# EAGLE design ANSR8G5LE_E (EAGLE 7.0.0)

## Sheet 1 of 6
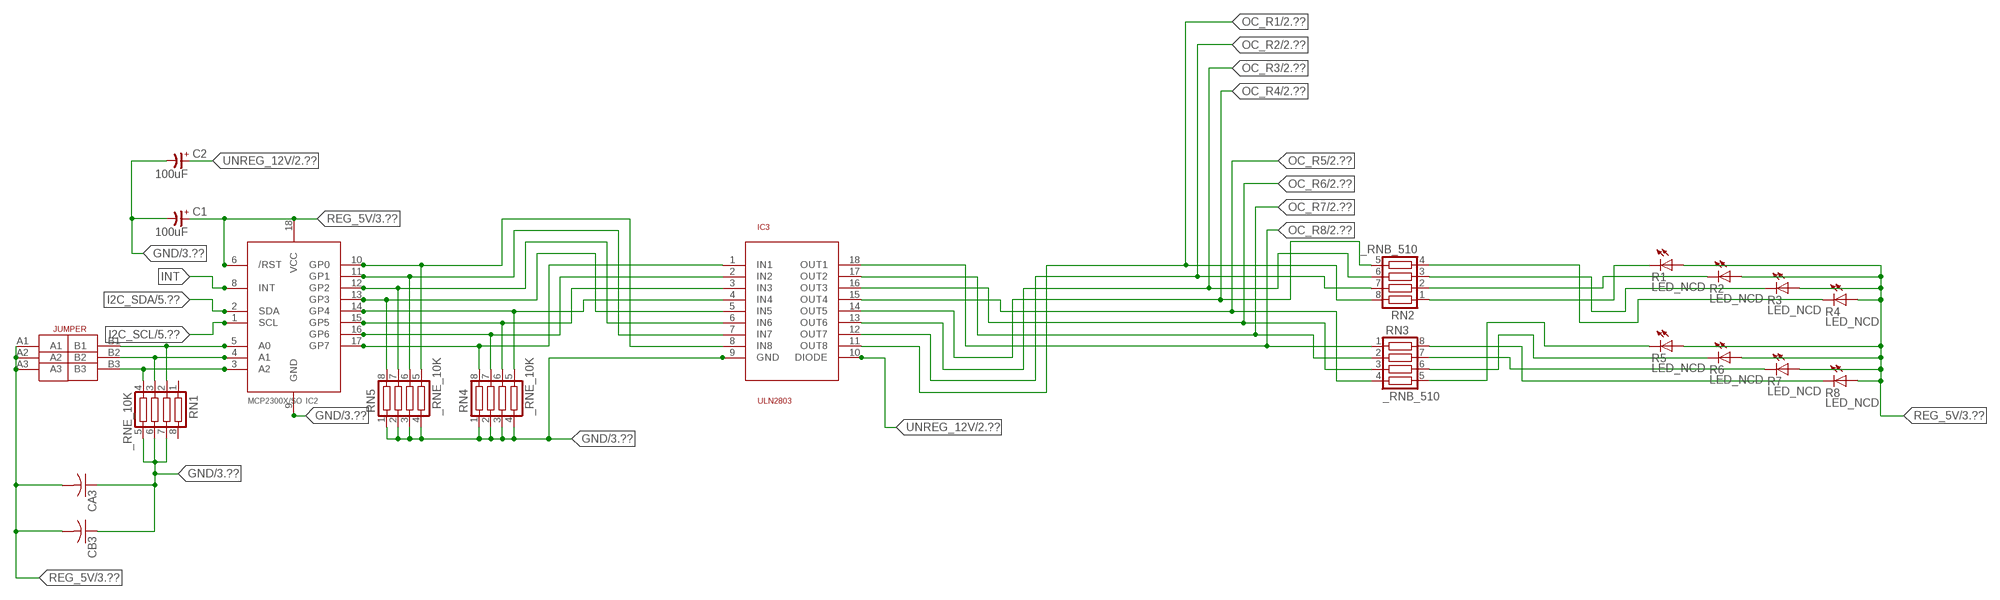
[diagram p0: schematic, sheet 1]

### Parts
C1  100uF  CP-E-025X060  [E-025X060]
C2  100uF  CP-E-025X060  [E-025X060]
CA3  CC1206KRX7R9BB104C1206K  [CC1206KRX7R9BB104]
CB3  TMK316F106ZL-TC1206K  [TMK316F106ZL-T]
IC2  MCP2300X/SO  [SO18W]
IC3  ULN2803  [SO18L]
R1  LED_NCD  [CHIPLED_0603]
R2  LED_NCD  [CHIPLED_0603]
R3  LED_NCD  [CHIPLED_0603]
R4  LED_NCD  [CHIPLED_0603]
R5  LED_NCD  [CHIPLED_0603]
R6  LED_NCD  [CHIPLED_0603]
R7  LED_NCD  [CHIPLED_0603]
R8  LED_NCD  [CHIPLED_0603]
RN1  _RNE_10K  [RNE]
RN2  _RNB_510  [RNB]
RN3  _RNB_510  [RNB]
RN4  _RNE_10K  [RNE]
RN5  _RNE_10K  [RNE]
U$18  JUMPER_3X2  [JUMPER_3X2]

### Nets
GND: C1.- C2.- CA3.1 CB3.1 IC2.9(GND) IC3.9(GND) RN1.5 RN1.6 RN1.7 RN4.1 RN4.2 RN4.3 RN4.4 RN5.1 RN5.2 RN5.3 RN5.4 ; also sheet 3,4,5,6
GP4: IC2.14(GP4) IC3.4(IN4) RN4.5
GP6: IC2.16(GP6) IC3.2(IN2) RN4.7
I2C_SCL: IC2.1(SCL) ; also sheet 5,6
I2C_SDA: IC2.2(SDA) ; also sheet 5,6
INT: IC2.8(INT)
N$6: IC2.5(A0) RN1.2 U$18.B1
N$7: IC2.4(A1) RN1.3 U$18.B2
N$8: IC2.3(A2) RN1.4 U$18.B3
N$20: R1.C RN2.1
N$21: IC2.12(GP2) IC3.6(IN6) RN5.7
N$22: IC2.11(GP1) IC3.7(IN7) RN5.6
N$23: IC2.10(GP0) IC3.8(IN8) RN5.5
N$29: R2.C RN2.2
N$30: R3.C RN2.3
N$31: R4.C RN2.4
N$32: R8.C RN3.8
N$81: R7.C RN3.7
N$82: R6.C RN3.6
N$83: R5.C RN3.5
N$89: IC2.13(GP3) IC3.5(IN5) RN5.8
N$93: IC2.15(GP5) IC3.3(IN3) RN4.6
N$94: IC2.17(GP7) IC3.1(IN1) RN4.8
OC_R1: IC3.11(OUT8) RN2.8 ; also sheet 2
OC_R2: IC3.12(OUT7) RN2.7 ; also sheet 2
OC_R3: IC3.13(OUT6) RN2.6 ; also sheet 2
OC_R4: IC3.14(OUT5) RN2.5 ; also sheet 2
OC_R5: IC3.15(OUT4) RN3.4 ; also sheet 2
OC_R6: IC3.16(OUT3) RN3.3 ; also sheet 2
OC_R7: IC3.17(OUT2) RN3.2 ; also sheet 2
OC_R8: IC3.18(OUT1) RN3.1 ; also sheet 2
REG_5V: C1.+ CA3.2 CB3.2 IC2.6(/RST) IC2.18(VCC) R1.A R2.A R3.A R4.A R5.A R6.A R7.A R8.A U$18.A1 U$18.A2 U$18.A3 ; also sheet 3,4,5,6
UNREG_12V: C2.+ IC3.10(DIODE) ; also sheet 2,3
Unconnected: RN1.1 RN1.8

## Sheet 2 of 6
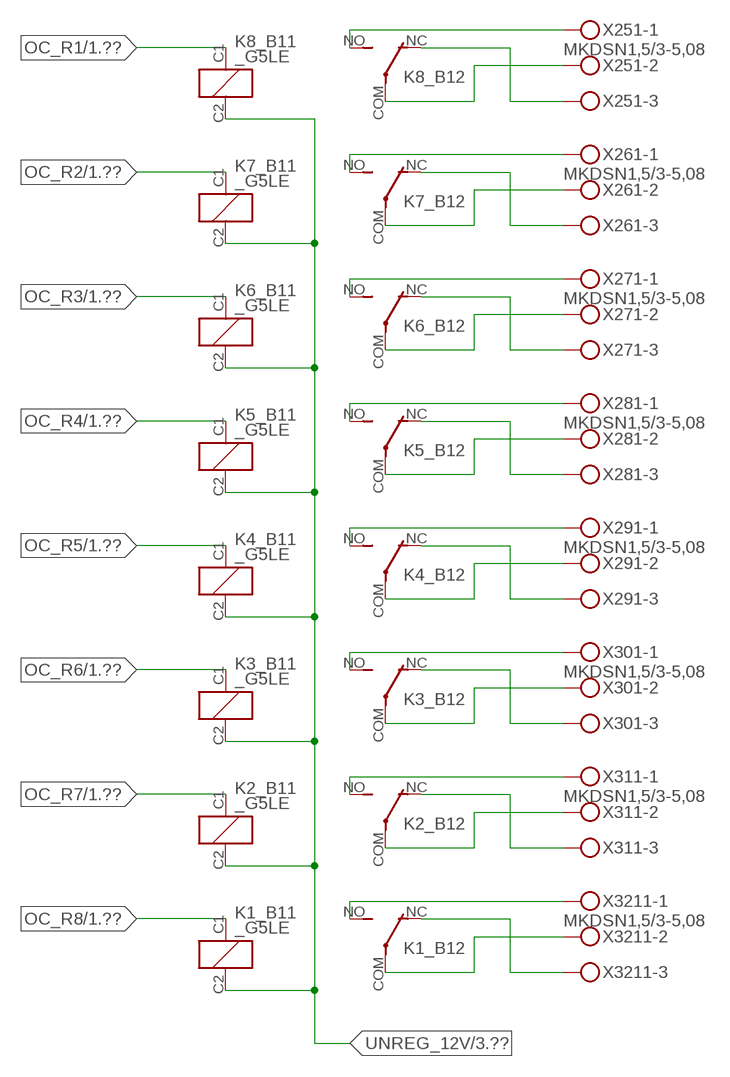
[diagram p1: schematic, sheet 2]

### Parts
K1_B1  _G5LE  [G5LE]
K2_B1  _G5LE  [G5LE]
K3_B1  _G5LE  [G5LE]
K4_B1  _G5LE  [G5LE]
K5_B1  _G5LE  [G5LE]
K6_B1  _G5LE  [G5LE]
K7_B1  _G5LE  [G5LE]
K8_B1  _G5LE  [G5LE]
X251  MKDSN1,5/3-5,08  [MKDSN1,5/3-5,08]
X261  MKDSN1,5/3-5,08  [MKDSN1,5/3-5,08]
X271  MKDSN1,5/3-5,08  [MKDSN1,5/3-5,08]
X281  MKDSN1,5/3-5,08  [MKDSN1,5/3-5,08]
X291  MKDSN1,5/3-5,08  [MKDSN1,5/3-5,08]
X301  MKDSN1,5/3-5,08  [MKDSN1,5/3-5,08]
X311  MKDSN1,5/3-5,08  [MKDSN1,5/3-5,08]
X3211  MKDSN1,5/3-5,08  [MKDSN1,5/3-5,08]

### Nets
N$203: K8_B1.COM(2:COM) X251.2
N$204: K8_B1.NC(2:NC) X251.3
N$205: K8_B1.NO(2:NO) X251.1
N$206: K7_B1.NO(2:NO) X261.1
N$207: K6_B1.NO(2:NO) X271.1
N$208: K7_B1.NC(2:NC) X261.3
N$209: K7_B1.COM(2:COM) X261.2
N$210: K6_B1.NC(2:NC) X271.3
N$211: K6_B1.COM(2:COM) X271.2
N$212: K5_B1.NC(2:NC) X281.3
N$213: K5_B1.COM(2:COM) X281.2
N$214: K5_B1.NO(2:NO) X281.1
N$215: K4_B1.NO(2:NO) X291.1
N$216: K4_B1.NC(2:NC) X291.3
N$217: K4_B1.COM(2:COM) X291.2
N$218: K3_B1.NO(2:NO) X301.1
N$219: K3_B1.NC(2:NC) X301.3
N$220: K3_B1.COM(2:COM) X301.2
N$221: K2_B1.NO(2:NO) X311.1
N$222: K2_B1.NC(2:NC) X311.3
N$223: K2_B1.COM(2:COM) X311.2
N$224: K1_B1.NO(2:NO) X3211.1
N$225: K1_B1.NC(2:NC) X3211.3
N$226: K1_B1.COM(2:COM) X3211.2
OC_R1: K8_B1.C1(1:C1) ; also sheet 1
OC_R2: K7_B1.C1(1:C1) ; also sheet 1
OC_R3: K6_B1.C1(1:C1) ; also sheet 1
OC_R4: K5_B1.C1(1:C1) ; also sheet 1
OC_R5: K4_B1.C1(1:C1) ; also sheet 1
OC_R6: K3_B1.C1(1:C1) ; also sheet 1
OC_R7: K2_B1.C1(1:C1) ; also sheet 1
OC_R8: K1_B1.C1(1:C1) ; also sheet 1
UNREG_12V: K1_B1.C2(1:C2) K2_B1.C2(1:C2) K3_B1.C2(1:C2) K4_B1.C2(1:C2) K5_B1.C2(1:C2) K6_B1.C2(1:C2) K7_B1.C2(1:C2) K8_B1.C2(1:C2) ; also sheet 1,3

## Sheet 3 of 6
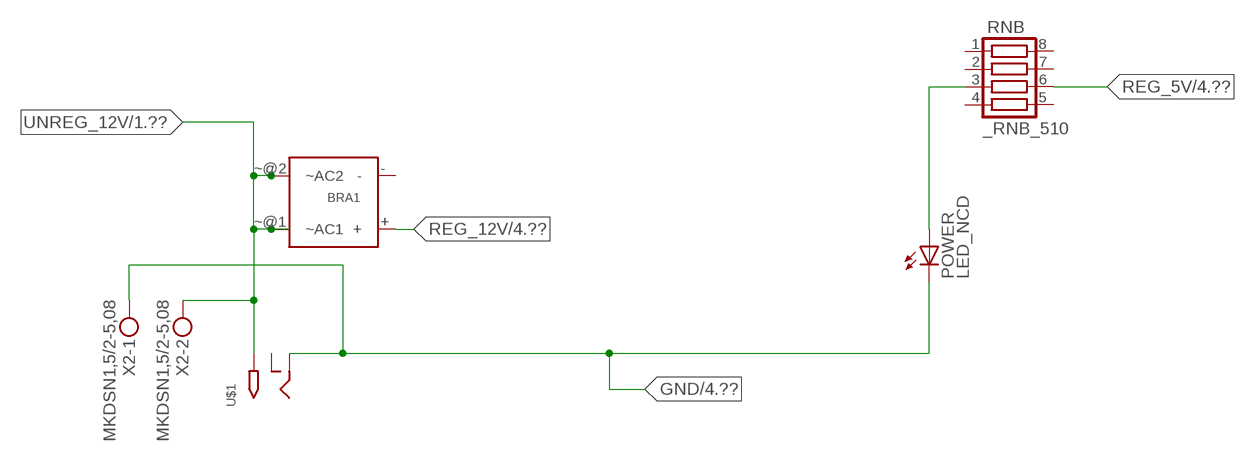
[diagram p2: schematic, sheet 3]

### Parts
BRA1  MB2S_  [MB2S]
POWER  LED_NCD  [CHIPLED_0603]
RNB  _RNB_510  [RNB]
U$1  2.1MMJACK  [PJ-102A]
X2  MKDSN1,5/2-5,08  [MKDSN1,5/2-5,08]

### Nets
GND: POWER.C U$1.RING X2.1 ; also sheet 1,4,5,6
N$2: POWER.A RNB.3
REG_5V: RNB.6 ; also sheet 1,4,5,6
REG_12V: BRA1.+ ; also sheet 4
UNREG_12V: BRA1.~@1(~AC1) BRA1.~@2(~AC2) U$1.TIP X2.2 ; also sheet 1,2
Unconnected: BRA1.- RNB.1 RNB.2 RNB.4 RNB.5 RNB.7 RNB.8 U$1.RING_SW

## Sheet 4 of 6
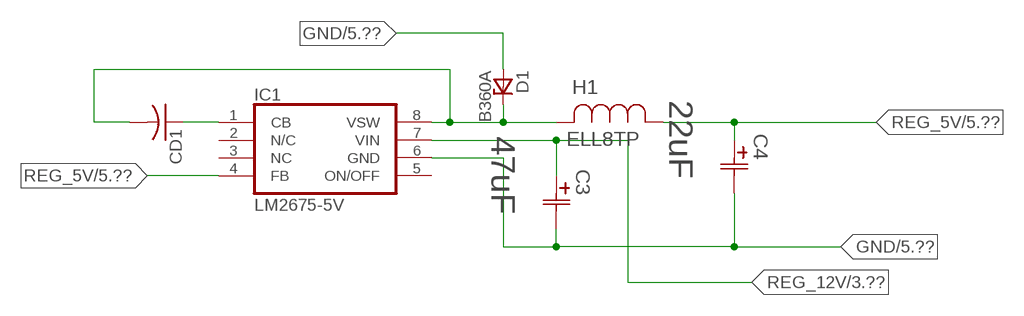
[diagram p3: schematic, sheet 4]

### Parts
C3  47uF  490-5463-6-NDCAP  [C2917(7343)-Y]
C4  22uF  490-5463-6-NDCAP  [C2917(7343)-Y]
CD1  _CD_10NF_50VC1206K  [_CD_10NF_50V]
D1  B360A  [DO214AC_ZENER]
H1  ELL8TP  [IND_ELL8TP]
IC1  LM2675-5V  LM2675  [SO-8]

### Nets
GND: C3.2(C2) C4.2(C2) D1.A IC1.6(GND) ; also sheet 1,3,5,6
N$1: CD1.2 D1.C H1.2 IC1.8(VSW)
N$3: CD1.1 IC1.1(CB)
REG_5V: C4.1(C1) H1.1 IC1.4(FB) ; also sheet 1,3,5,6
REG_12V: C3.1(C1) IC1.7(VIN) ; also sheet 3
Unconnected: IC1.2(N/C) IC1.5(ON/OFF)

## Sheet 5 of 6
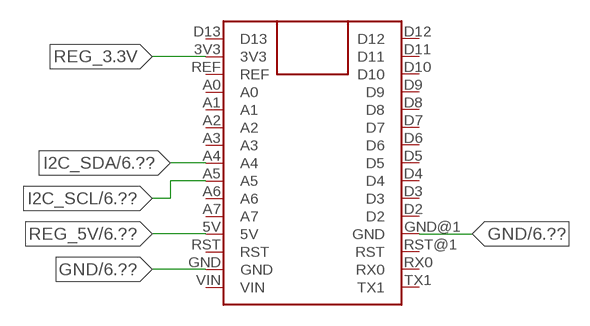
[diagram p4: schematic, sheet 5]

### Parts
FOR_NANO  ARDUINO_NANO  [ARDUINO_NANO]

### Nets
GND: FOR_NANO.GND FOR_NANO.GND@1(GND) ; also sheet 1,3,4,6
I2C_SCL: FOR_NANO.A5 ; also sheet 1,6
I2C_SDA: FOR_NANO.A4 ; also sheet 1,6
REG_3.3V: FOR_NANO.3V3
REG_5V: FOR_NANO.5V ; also sheet 1,3,4,6
Unconnected: FOR_NANO.A0 FOR_NANO.A1 FOR_NANO.A2 FOR_NANO.A3 FOR_NANO.A6 FOR_NANO.A7 FOR_NANO.D2 FOR_NANO.D3 FOR_NANO.D4 FOR_NANO.D5 FOR_NANO.D6 FOR_NANO.D7 FOR_NANO.D8 FOR_NANO.D9 FOR_NANO.D10 FOR_NANO.D11 FOR_NANO.D12 FOR_NANO.D13 FOR_NANO.REF FOR_NANO.RST FOR_NANO.RST@1(RST) FOR_NANO.RX0 FOR_NANO.TX1 FOR_NANO.VIN

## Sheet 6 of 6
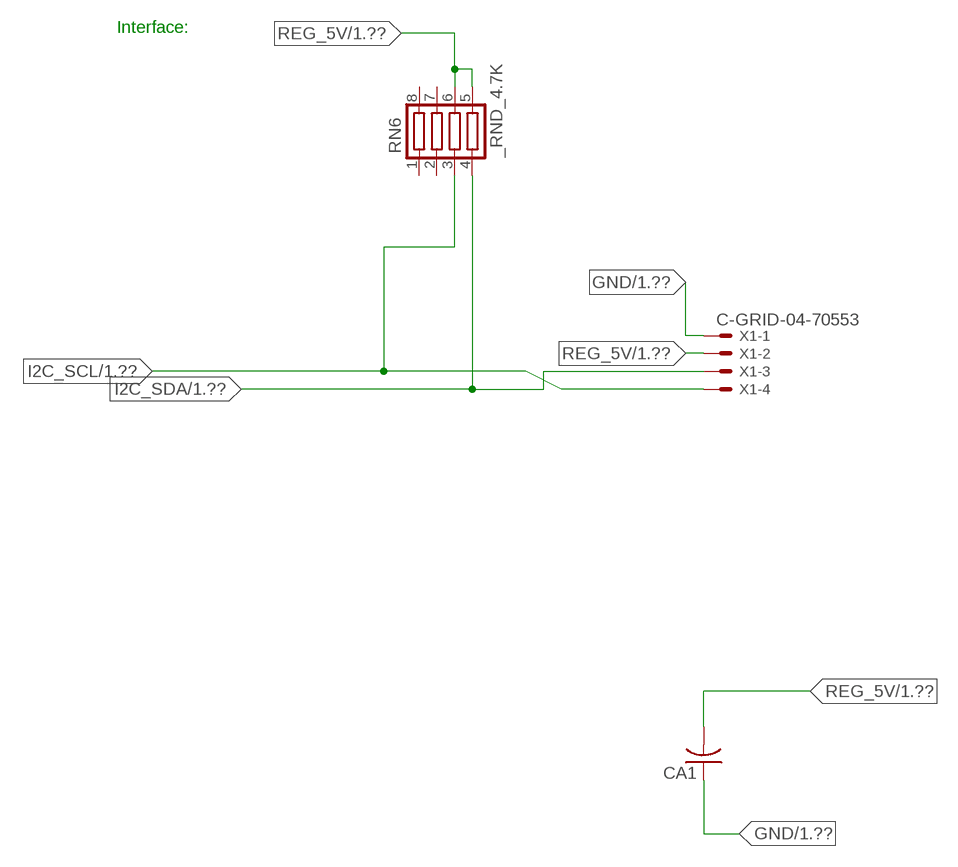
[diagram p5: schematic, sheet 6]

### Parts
CA1  CC1206KRX7R9BB104  [.1UF]
RN6  _RND_4.7K  [RND]
X1  C-GRID-04-70553  [70553-04]

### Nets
GND: CA1.1 X1.1 ; also sheet 1,3,4,5
I2C_SCL: RN6.3 X1.4 ; also sheet 1,5
I2C_SDA: RN6.4 X1.3 ; also sheet 1,5
REG_5V: CA1.2 RN6.5 RN6.6 X1.2 ; also sheet 1,3,4,5
Unconnected: RN6.1 RN6.2 RN6.7 RN6.8

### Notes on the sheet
- Interface:

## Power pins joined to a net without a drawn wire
NC: IC1.3(NC)

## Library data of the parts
BRA1 = NCD_ULTIMATE_LIBRARY:MB2S: Bridge Rectifier BRA MB2S 200V 500ma Digikey MB2S-TPMSTR-ND/MB2S-TP
C1 C2 = NCD_ULTIMATE_LIBRARY:CP-: Capacitors All Kinds POLARIZED CAP
C3 C4 = NCD_ULTIMATE_bhaskar:490-5463-6-ND: NCD CAP
CA1 CA3 = NCD_ULTIMATE_LIBRARY:CC1206KRX7R9BB104: Capacitor CA .1uF 50V SMT C1206K CC1206KRX7R9BB104
CB3 = NCD_ULTIMATE_LIBRARY:TMK316F106ZL-T: Capacitor CB 10uF SMT 1206 TMK316F106ZL-T
CD1 = NCD_ULTIMATE_LIBRARY:_CD_10NF_50V: Capacitor 10nF SMT
D1 = NCD_ULTIMATE_bhaskar:B360A: NCD DIODE B350A/B360A
FOR_NANO = NCD_ULTIMATE_CONNECTORS:ARDUINO_NANO
H1 = NCD_ULTIMATE_bhaskar:ELL8TP: NCD coil
IC1 = NCD_ULTIMATE_bhaskar:LM2675: LM2675 NCD http://www.ti.com/lit/ds/symlink/lm2675.pdf
IC2 = NCD_ULTIMATE_LIBRARY:MCP2300X: Semiconductor Port Expander I/O 8-Bit I2C MCP23008 Inexpensive i2c i/o expander - 8 general purpose i/o pins with optional pullups
IC3 = NCD_ULTIMATE_LIBRARY:ULN2803: Semiconductor 8 O.C. N-Channel Transistor Driver Digikey ULN2803AFWGCELTR-ND/ULN2803AFWG,C,EL
K1_B1 K2_B1 K3_B1 K4_B1 K5_B1 K6_B1 K7_B1 K8_B1 = NCD_ULTIMATE_LIBRARY:_G5LE: Relay 5A/10A SPDT; OC_FARNELL: unknown; OC_NEWARK: unknown
POWER = NCD_ULTIMATE_bhaskar:LED_NCD
R1-R8 = NCD_ULTIMATE_LIBRARY:LED_NCD: LED Digikey 754-1132-2-ND/APT2012SRCPRV
RN1 RN4 RN5 = NCD_ULTIMATE_LIBRARY:_RNE_10K: Resistor Array RNE SMT 10K x 4 Single Resistor Source: http://www.ctscorp.com/components/Datasheets/CTSChipArrayDs.pdf Digikey 742C083103JPTR-ND/742C083103JP; OC_FARNELL: unknown; OC_NEWARK: unknown
RN2 RN3 RNB = NCD_ULTIMATE_LIBRARY:_RNB_510: Resistor Array RNB SMT 510 x 4 Single Resistor Source: http://www.ctscorp.com/components/Datasheets/CTSChipArrayDs.pdf Digikey 742C083511JPTR-ND/ 742C083511JP; OC_FARNELL: unknown; OC_NEWARK: unknown
RN6 = NCD_ULTIMATE_LIBRARY:_RND_4.7K: Resistor Array RND SMT 4.7K x 4 Single Resistor Source: http://www.ctscorp.com/components/Datasheets/CTSChipArrayDs.pdf Digikey 742C083472JPTR-ND/742C083472JP; OC_FARNELL: unknown; OC_NEWARK: unknown
U$1 = NCD_ULTIMATE_CONNECTORS:2.1MMJACK: 2.1mm x 5.5mm DC jack with internal switch. Digikey part #PJ-102A, 4UCON part #05537 By microbuilder.eu
U$18 = NCD_ULTIMATE_CONNECTORS:JUMPER_3X2
X1 = NCD_ULTIMATE_CONNECTORS:C-GRID-04: CONNECTOR 4-Pos I2C wire to board 2.54 mm (0.100") pitch header Digikey WM1342-ND/0015912045; OC_FARNELL: unknown; OC_NEWARK: unknown
X2 = NCD_ULTIMATE_CONNECTORS:MKDSN1,5/2-5,08: MKDSN 1,5/ 2-5,08 Printklemme
X251 X261 X271 X281 X291 X301 X311 X3211 = NCD_ULTIMATE_CONNECTORS:MKDSN1,5/3-5,08: MKDSN 1,5/ 3-5,08 Printklemme Nennstrom: 13,5 A Nennspannung: 250 V Rastermaß: 5,08 mm Polzahl: 3 Anschlussart: Schraubanschluss Montage: Löten Anschlussrichtung Leiter/Platine: 0 ° Artikelnummer: 1729131 Source: http://eshop.phoenixcontact.com .. 1729131.pdf

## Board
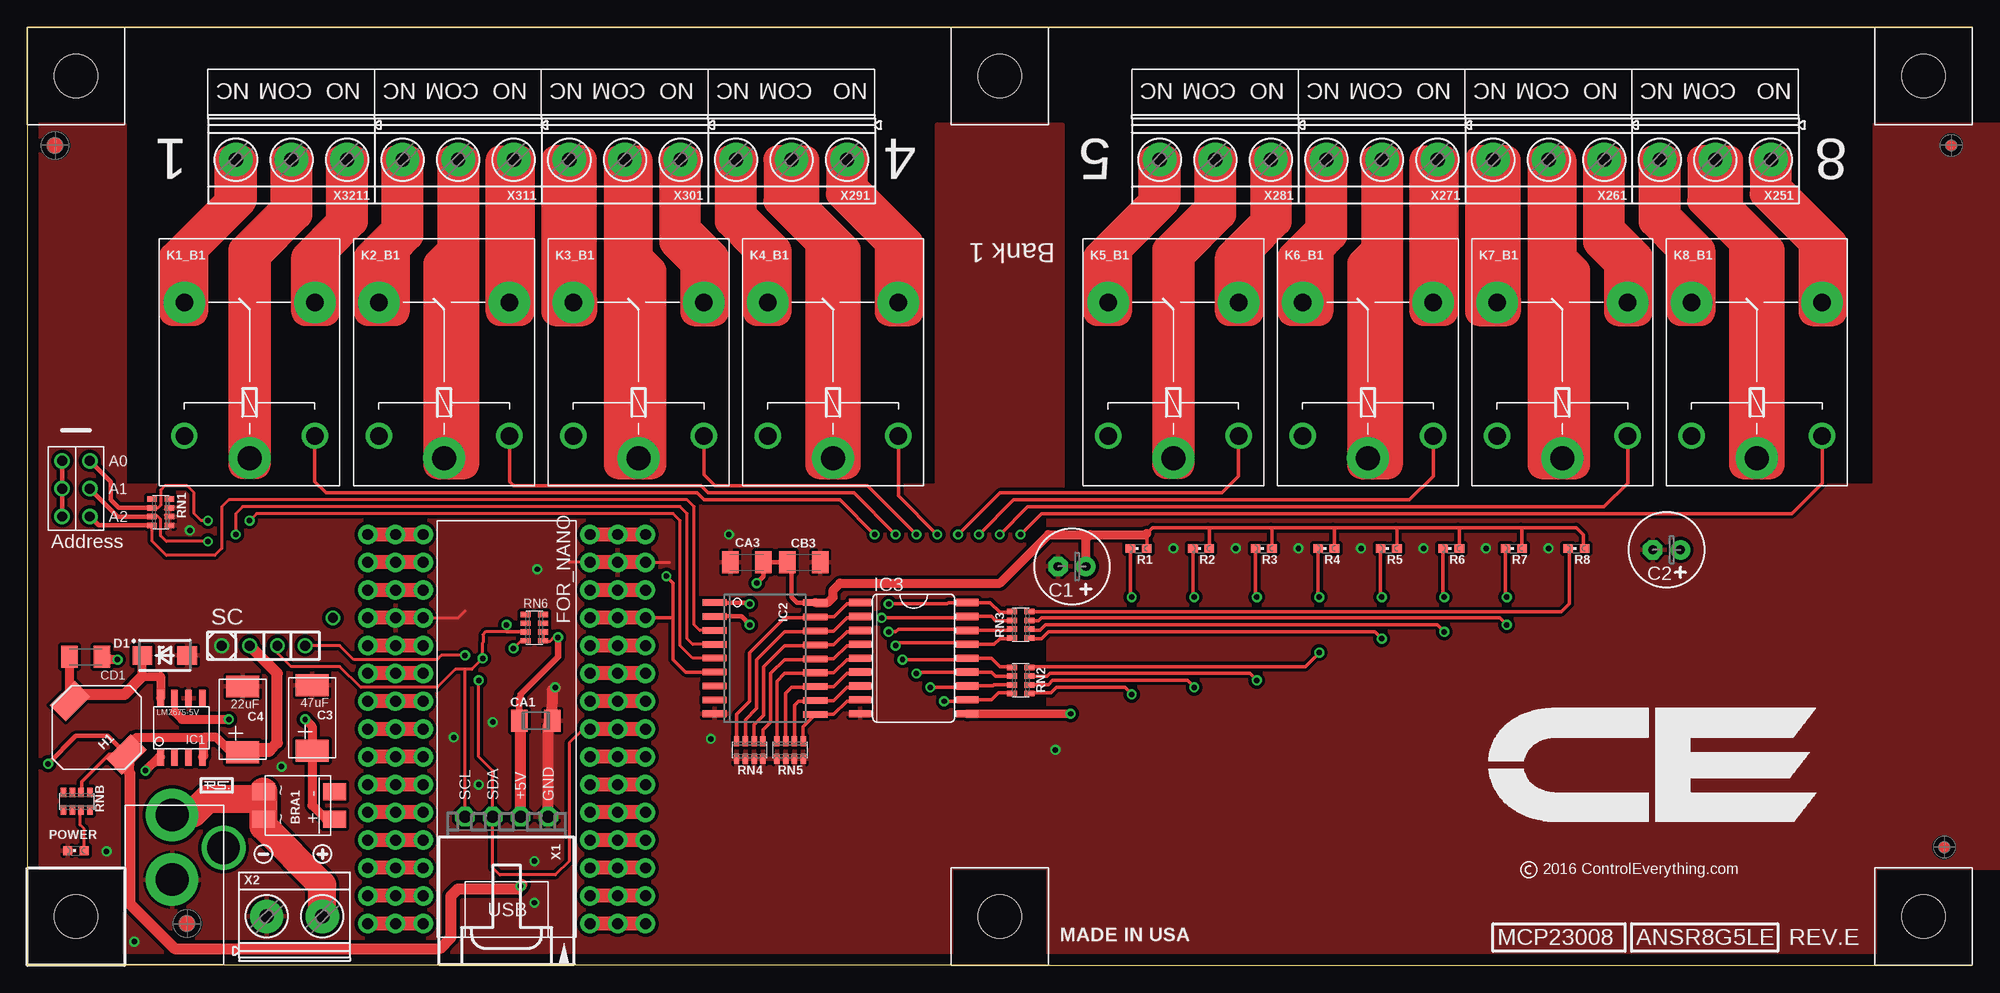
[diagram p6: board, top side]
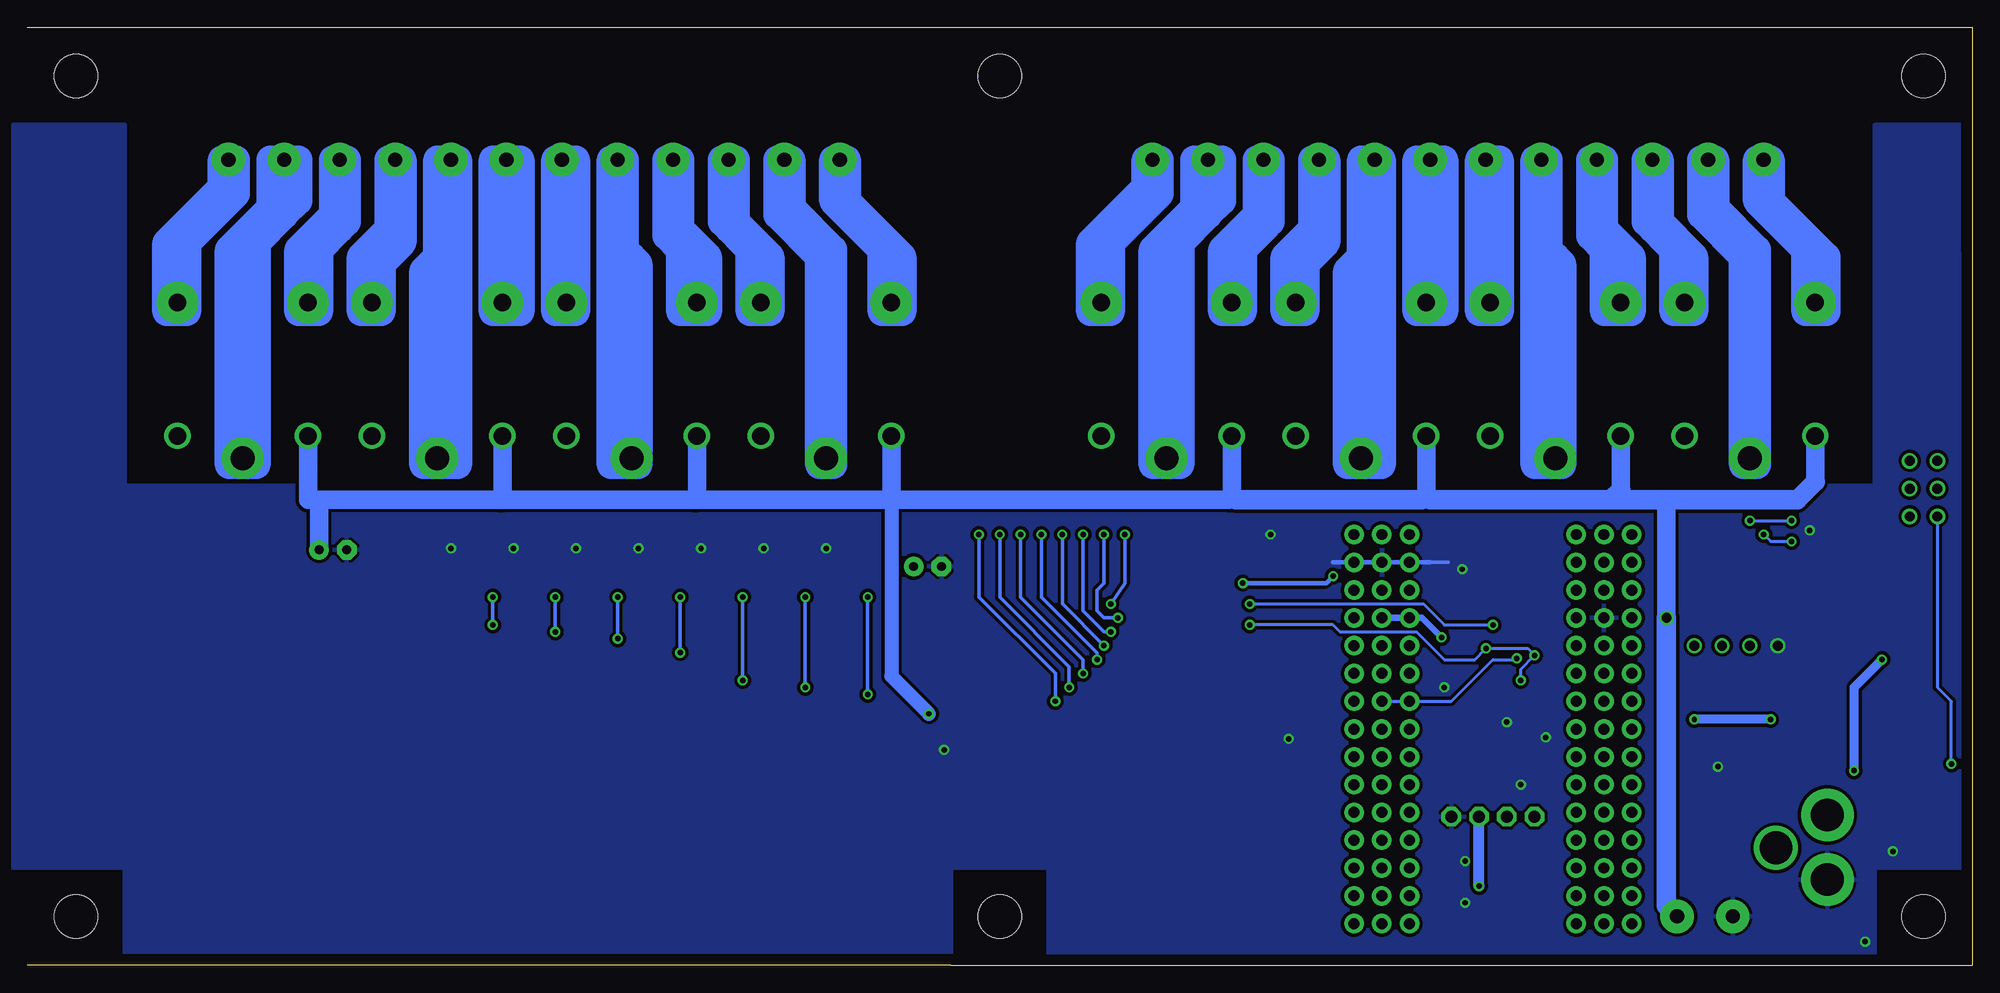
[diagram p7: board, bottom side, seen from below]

Size 177.8 x 85.73 mm. Coordinates in mm from the lower left corner, seen from the top.
Outline: 0,66.34 0,65.41
Outline: 0,65.41 0,0 93.34,0 177.8,0
Outline: 177.8,85.73 0,85.73 0,65.41
Copper layers (1*16): Top 0.035mm / dielectric 1.5mm / Bottom 0.035mm
Design rules "default": minimum track width 10mil, minimum drill 24mil, track to track 8mil, track to pad 8mil, pad to pad 8mil, via to via 8mil, smd to smd 8mil, copper to edge 40mil, drill to drill 8mil, minimum pad ring 10mil, minimum via ring 8mil, stop-mask expansion 4mil, vias tented up to drill 0mil, thermal gap 10mil
Holes 3.96 mm at 4.45,4.45 4.45,4.45 4.45,4.45 4.45,4.45

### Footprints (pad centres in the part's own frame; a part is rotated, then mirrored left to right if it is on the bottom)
MB2S = smd 1.55 x 2.1: + 0,-6.5; - 2.54,-6.5; ~@1 0,0; ~@2 2.54,0
E-025X060 = drill 0.813 pad 1.778: + -1.27,0 | drill 0.813 pad 1.778 octagon: - 1.27,0
C2917(7343)-Y = smd 2 x 3: 1 -3,0; 2 3,0
.1UF = smd 1.5 x 2: 1 -1.5,0; 2 1.5,0
CC1206KRX7R9BB104 = smd 1.5 x 2: 1 -1.5,0; 2 1.5,0
TMK316F106ZL-T = smd 1.5 x 2: 1 -1.5,0; 2 1.5,0
_CD_10NF_50V = smd 1.5 x 2: 1 -1.5,0; 2 1.5,0
DO214AC_ZENER = smd 1.8 x 1.7: A 2.05,0; C -2.05,0
ARDUINO_NANO = drill 1 pad 1.778: 3V1 -2.54,-2.54; 3V3 0,-2.54; 5V 0,-27.94; 5V1 -2.54,-27.94; A0 0,-7.62; A1 0,-10.16; A2 0,-12.7; A3 0,-15.24; A4 0,-17.78; A5 0,-20.32; A6 0,-22.86; A7 0,-25.4; A8 -2.54,-7.62; A9 -2.54,-10.16; A10 -2.54,-12.7; A11 -2.54,-15.24; A12 -2.54,-17.78; A13 -2.54,-20.32; A14 -2.54,-22.86; A15 -2.54,-25.4; D1 -2.54,0; D2 20.32,-25.4; D3 20.32,-22.86; D4 20.32,-20.32; D5 20.32,-17.78; D6 20.32,-15.24; D7 20.32,-12.7; D8 20.32,-10.16; D9 20.32,-7.62; D10 20.32,-5.08; D11 20.32,-2.54; D12 20.32,0; D13 0,0; D14 22.86,0; D15 22.86,-2.54; D16 22.86,-5.08; D17 22.86,-7.62; D18 22.86,-10.16; D19 22.86,-12.7; D20 22.86,-15.24; D21 22.86,-17.78; D22 22.86,-20.32; D23 22.86,-22.86; D24 22.86,-25.4; GND 0,-33.02; GND1 -2.54,-33.02; GND@1 20.32,-27.94; GND@2 22.86,-27.94; P$16 2.54,0; P$17 2.54,-2.54; P$18 2.54,-5.08; P$19 2.54,-7.62; P$20 2.54,-10.16; P$21 2.54,-12.7; P$22 2.54,-15.24; P$23 2.54,-17.78; P$24 2.54,-20.32; P$25 2.54,-22.86; P$26 2.54,-25.4; P$27 2.54,-27.94; P$28 2.54,-30.48; P$29 2.54,-33.02; P$30 2.54,-35.56; P$31 17.78,0; P$32 17.78,-2.54; P$33 17.78,-5.08; P$34 17.78,-7.62; P$35 17.78,-10.16; P$36 17.78,-12.7; P$37 17.78,-15.24; P$38 17.78,-17.78; P$39 17.78,-20.32; P$40 17.78,-22.86; P$41 17.78,-25.4; P$42 17.78,-27.94; P$43 17.78,-30.48; P$44 17.78,-33.02; P$45 17.78,-35.56; REF 0,-5.08; REF1 -2.54,-5.08; RST 0,-30.48; RST1 -2.54,-30.48; RST@1 20.32,-30.48; RST@2 22.86,-30.48; RX0 20.32,-33.02; RX1 22.86,-33.02; TX1 20.32,-35.56; TX2 22.86,-35.56; VIN 0,-35.56; VIN1 -2.54,-35.56
IND_ELL8TP = smd 2.054 x 3.2 rotated 45: 1 -2.442,-2.696; 2 2.442,2.442
SO-8 = smd 0.6 x 1.55: 1 -1.905,-2.69; 2 -0.635,-2.69; 3 0.635,-2.69; 4 1.905,-2.69; 5 1.905,2.71; 6 0.635,2.71; 7 -0.635,2.71; 8 -1.905,2.71
SO18W = smd 0.6 x 2.2: 1 -4.445,-4.6; 2 -3.175,-4.6; 3 -1.905,-4.6; 4 -0.635,-4.6; 5 0.635,-4.6; 6 1.905,-4.6; 7 3.175,-4.6; 8 4.445,-4.6; 9 5.715,-4.6; 10 5.775,4.6; 11 4.505,4.6; 12 3.235,4.6; 13 1.965,4.6; 14 0.695,4.6; 15 -0.575,4.6; 16 -1.845,4.6; 17 -3.145,4.6; 18 -4.445,4.6
SO18L = smd 0.66 x 2.032: 1 -5.08,-4.902; 2 -3.81,-4.902; 3 -2.54,-4.902; 4 -1.27,-4.902; 5 0,-4.902; 6 1.27,-4.902; 7 2.54,-4.902; 8 3.81,-4.902; 9 5.08,-4.902; 10 5.08,4.902; 11 3.81,4.902; 12 2.54,4.902; 13 1.27,4.902; 14 0,4.902; 15 -1.27,4.902; 16 -2.54,4.902; 17 -3.81,4.902; 18 -5.08,4.902
G5LE = drill 1.6: C1 -7.493,-5.969; C2 -7.493,5.969 | drill 2.2 pad 3.81: COM -9.525,0 | drill 1.6 pad 3.81: NC 4.699,5.969; NO 4.699,-5.969
CHIPLED_0603 = smd 0.8 x 0.8: A 0,-0.75; C 0,0.75
CHIPLED_0603' = smd 0.8 x 0.876: A 0,-0.75; C 0,0.75
RNE = smd 0.5 x 0.9: 1 -1.2,-0.8; 2 -0.4,-0.8; 3 0.4,-0.8; 4 1.2,-0.8; 5 1.2,0.8; 6 0.4,0.8; 7 -0.4,0.8; 8 -1.2,0.8
RNB = smd 0.5 x 0.9: 1 -1.2,-0.8; 2 -0.4,-0.8; 3 0.4,-0.8; 4 1.2,-0.8; 5 1.2,0.8; 6 0.4,0.8; 7 -0.4,0.8; 8 -1.2,0.8
RND = smd 0.5 x 0.9: 1 -1.2,-0.8; 2 -0.4,-0.8; 3 0.4,-0.8; 4 1.2,-0.8; 5 1.2,0.8; 6 0.4,0.8; 7 -0.4,0.8; 8 -1.2,0.8
PJ-102A = drill 3 pad 4.8: RING 0.1,-3.39; TIP 0.1,-9.29 | drill 3 pad 3.251: RING_SW -4.6,-6.29
PCB_MOUNTING_HOLE = hole 3.962: 4.445,4.445
JUMPER_3X2 = drill 0.9: A1 0,5.08; A2 0,2.54; A3 0,0; B1 2.54,5.08; B2 2.54,2.54; B3 2.54,0
70553-04 = drill 1.1 pad 1.778 octagon: 1 -3.81,-7.62; 2 -1.27,-7.62; 3 1.27,-7.62; 4 3.81,-7.62
MKDSN1,5/2-5,08 = drill 1.3 pad 3.048: 1 -2.561,0.025; 2 2.519,0.025
MKDSN1,5/3-5,08 = drill 1.3 pad 3.048: 1 -7.641,0.025; 2 -2.561,0.025; 3 2.519,0.025

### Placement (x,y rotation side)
BRA1  21.59,13.34 90 top
C1  95.5,36.45 180 top
C2  149.86,37.97 180 top
C3  26.04,22.61 90 top
C4  19.68,22.48 90 top
CA1  46.48,22.35 180 top
CA3  65.79,36.83 0 top
CB3  70.99,36.83 180 top
CD1  5.33,28.19 180 top
D1  12.57,28.32 0 top
FOR_NANO  53.98,3.81 180 top
H1  6.35,21.72 90 top
IC1  14.1,21.72 0 top
IC2  67.44,28.7 270 top
IC3  81.03,28.07 270 top
K1_B1  20.32,55.88 90 top
K2_B1  38.1,55.88 90 top
K3_B1  55.88,55.88 90 top
K4_B1  73.66,55.88 90 top
K5_B1  104.78,55.88 90 top
K6_B1  122.56,55.88 90 top
K7_B1  140.34,55.88 90 top
K8_B1  158.12,55.88 90 top
POWER  4.45,10.48 90 top
R1  LED_NCD  [CHIPLED_0603']  101.6,38.1 90 top
R2  LED_NCD  [CHIPLED_0603']  107.31,38.1 90 top
R3  LED_NCD  [CHIPLED_0603']  113.03,38.1 90 top
R4  LED_NCD  [CHIPLED_0603']  118.75,38.1 90 top
R5  LED_NCD  [CHIPLED_0603']  124.46,38.1 90 top
R6  LED_NCD  [CHIPLED_0603']  130.18,38.1 90 top
R7  LED_NCD  [CHIPLED_0603']  135.89,38.1 90 top
R8  LED_NCD  [CHIPLED_0603']  141.6,38.1 90 top
RN1  12.19,41.4 270 top
RN2  90.81,26.04 90 top
RN3  90.81,31.12 270 top
RN4  66.04,19.69 0 top
RN5  69.72,19.69 0 top
RN6  46.35,30.86 270 top
RNB  4.51,14.99 0 top
U$1  13.34,4.45 180 top
U$2  [VISION_REF15]  14.61,3.81 0 top
U$3  [ICON_MINUS]  21.59,10.16 180 top
U$4  [VISION_REF10]  175.26,10.79 270 top
U$5  PCB_MOUNTING_HOLE  [PCB_MOUNTING_HOLE]  177.8,76.84 90 top
U$6  PCB_MOUNTING_HOLE  [PCB_MOUNTING_HOLE]  93.34,0 90 top
U$7  PCB_MOUNTING_HOLE  [PCB_MOUNTING_HOLE]  93.34,76.84 90 top
U$8  PCB_MOUNTING_HOLE  [PCB_MOUNTING_HOLE]  8.89,76.84 90 top
U$9  [ICON_PLUS]  26.99,10.16 90 top
U$11  PCB_MOUNTING_HOLE  [PCB_MOUNTING_HOLE]  177.8,0 90 top
U$12  PCB_MOUNTING_HOLE  [PCB_MOUNTING_HOLE]  177.8,76.84 90 top
U$15  [VISION_REF15]  2.54,74.93 270 top
U$18  3.17,41.02 0 top
U$21  [ICON_USA]  94.36,2.16 0 top
U$28  [VISION_REF10]  175.9,74.93 270 top
X1  43.81,5.97 180 top
X2  24.45,4.45 0 top
X251  151.76,73.66 180 top
X261  136.53,73.66 180 top
X271  121.28,73.66 180 top
X281  106.05,73.66 180 top
X291  67.31,73.66 180 top
X301  52.07,73.66 180 top
X311  36.83,73.66 180 top
X3211  21.59,73.66 180 top

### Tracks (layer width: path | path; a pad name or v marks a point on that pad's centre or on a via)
GND  (via drill 0.5, 0.9)
  Top 0.254: 36.2,31.75 39.37,31.75 40.01,32.38 | FOR_NANO.GND@1 32.38,31.75 | 49.53,36.83 56.52,36.83 58.67,36.83
  Top 1.016: X1.1 47.62,22 CA1.1 47.98,22.5 48.01,25.15 v48.26,25.4
  Bottom 0.254: 51.44,36.83 FOR_NANO.GND
  Bottom 0.305: 47.88,36.83 49.53,36.83 51.44,36.83
  Bottom 0.406: 49.53,36.83 58.42,36.83
  other vias: 14.86,39.75 62.48,20.7 127.64,38.1 93.98,19.69 133.35,38.1 139.06,38.1 121.92,38.1 116.2,38.1 110.49,38.1 104.78,38.1 64.14,39.37 9.78,2.16 17.78,29.21 41.27,16.51 46.35,9.53 46.61,36.2 46.35,5.71 42.55,22.23 38.99,20.83 7.24,10.41 23.24,18.16
  pour Bottom (isolate 0.305): -1.27,8.89 8.89,8.89 8.89,0 84.45,0 84.45,8.89 94.61,8.89 94.61,76.84 83.19,76.84 83.19,43.81 8.89,43.81 8.89,76.84 -1.27,76.84
  pour Top (isolate 0.305): -2.54,8.89 8.89,8.89 8.89,0 84.45,0 84.45,8.89 94.61,8.89 94.61,76.84 83.19,76.84 83.19,43.81 8.89,43.81 8.89,76.84 -2.54,76.84
  pour Top (isolate 0.305): 93.34,43.81 168.91,43.81 168.91,76.84 180.97,76.84 180.97,8.89 168.91,8.89 168.91,0 93.34,0
  pour Bottom (isolate 0.305): 93.34,0 93.34,43.81 168.91,43.81 168.91,76.84 179.07,76.84 179.07,8.89 168.91,8.89 168.91,0
GP4
  Top 0.305: RN4.5 67.24,21.52 67.94,22.23 67.94,26.67 69.22,27.94 71.97,27.94 IC2.14 73.73,28.01 74.93,29.21 76,29.21 IC3.4
GP6
  Top 0.305: RN4.7 65.64,22.46 66.67,23.5 66.67,27.94 69.22,30.48 71.97,30.48 IC2.16 73.73,30.55 74.93,31.75 76,31.75 IC3.2
I2C_SCL  (via drill 0.5, 0.9)
  Top 0.254: 40.01,27.05 40.64,27.05 v41.64,28.05 41.64,29.48 41.66,29.5 41.66,30.23 41.89,30.46 RN6.3 45.54,30.48 43.81,30.48 v43.81,31.12 | 40.01,27.05 39.12,27.05 37.47,25.4 30.48,25.4 28.57,27.3 24.13,27.3 22.86,28.58 v22.86,29.21 | X1.4 40.01,27.05
  Top 0.406: IC2.1 65.91,33.15 v66.04,33.02
  Bottom 0.254: v66.04,33.02 50.16,33.02 48.26,31.12 v43.81,31.12 | v41.64,28.05 41.75,27.94 43.81,27.94 47.62,24.13 FOR_NANO.A5
I2C_SDA  (via drill 0.5, 0.9)
  Top 0.254: RN6.4 45.16,29.66 v44.45,28.96 | 40,28.33 v40.01,28.32 37.85,28.32 37.47,27.94 29.84,27.94 28.57,29.21 v25.4,29.21 | v41.27,26.04 41.27,19.05 42.55,17.78 X1.3 42.55,8.89 43.18,8.26 48.26,8.26 49.53,9.53 49.53,20.32 50.8,21.59 51.44,21.59
  Top 0.406: IC2.2 65.28,31.88 v66.04,31.12
  Bottom 0.254: v66.04,31.12 58.42,31.12 57.78,30.48 50.8,30.48 48.26,27.94 45.47,27.94 v44.45,28.96 40.64,28.96 v40.01,28.32 41.27,27.05 v41.27,26.04
N$1
  Top 0.813: H1.2 3.88,24.77 | D1.C 10.52,26.4 12.19,26.38 IC1.8 | CD1.2 3.83,24.15 4.45,24.77
  Top 1.016: 3.88,24.77 4.45,24.77 8.89,24.77 10.52,26.4
N$2
  Top 0.254: POWER.A 5.2,12.46 4.83,12.83 4.83,14.1 RNB.3
  Top 0.406: 4.95,14.14 RNB.3
N$3  (via drill 0.5)
  Top 0.813: IC1.1 12.04,19.03 v10.79,17.78 | v8.26,27.94 7.72,27.94 CD1.1
  Bottom 0.813: v10.79,17.78 10.79,25.4 v8.26,27.94
N$6  (via drill 0.5)
  Top 0.254: IC2.5 60.83,28.07 59.69,29.21 59.69,40.64 59.05,41.27 20.95,41.27 v20.32,40.64 | v16.51,40.64 15.88,40.64 15.24,41.27 15.24,43.18 14.61,43.81 12.57,43.81 12.19,43.43 12.19,42.04 11.94,41.78 11.41,41.78 RN1.2
  Top 0.406: RN1.2 8.36,41.8 7.62,42.55 7.62,44.2 U$18.B1
  Bottom 0.254: v20.32,40.64 v16.51,40.64
N$7  (via drill 0.5)
  Top 0.254: IC2.4 60.83,29.34 60.33,29.84 60.33,41.27 59.69,41.91 19.68,41.91 19.05,41.27 v19.05,39.37 | v16.51,38.73 12.7,38.73 12.19,39.24 12.19,40.77 11.94,41.02 11.41,41.02 RN1.3
  Top 0.406: RN1.3 8.27,41 U$18.B2
  Bottom 0.254: v19.05,39.37 18.41,38.73 v16.51,38.73
N$8
  Top 0.254: IC2.3 61.47,30.61 60.96,31.12 60.96,41.91 60.33,42.55 18.41,42.55 17.78,41.91 17.78,38.1 17.14,37.47 12.7,37.47 11.43,38.73 11.43,40.16 RN1.4
  Top 0.406: RN1.4 6.53,40.2 U$18.B3
N$9
  Top 2.54: 74.95,73.64 74.95,70.46 79.38,66.04 79.38,60.83 79.63,60.58
N$10
  Top 2.54: 64.79,73.64 64.79,68.56 67.31,66.04 67.31,60.96 67.69,60.58
N$11
  Top 2.54: 69.87,73.64 69.87,69.83 73.66,66.04 73.66,46.35
N$12
  Top 2.54: 59.71,73.64 59.71,66.02 61.59,64.14 61.59,60.83 61.85,60.58
N$13
  Top 2.54: 49.55,73.64 49.55,60.94 49.91,60.58
N$14
  Top 2.54: 54.63,73.64 54.63,47.6 55.88,46.35
N$15
  Top 2.54: 44.47,73.64 44.47,60.98 44.07,60.58
N$16
  Top 2.54: 34.31,73.64 34.31,66.7 32.38,64.77 32.38,60.83 32.13,60.58
N$17
  Top 2.54: 39.39,73.64 39.39,47.65 38.1,46.35
N$18
  Top 2.54: 29.23,73.64 29.23,67.97 26.67,65.41 26.67,60.96 26.29,60.58
N$19
  Top 2.54: 19.07,73.64 19.07,69.87 14.61,65.41 14.61,60.83 14.35,60.58
N$20  (via drill 0.5)
  Top 0.305: R1.C 100.85,33.77 v100.97,33.66 | v100.97,24.77 100.33,25.4 94.11,25.4 93.6,24.89 91.66,24.89 RN2.1
  Bottom 0.305: v100.97,33.66 v100.97,24.77
N$21
  Top 0.305: RN5.7 69.32,24.87 69.85,25.4 71.97,25.4 IC2.12 73.73,25.47 74.93,26.67 76,26.67 IC3.6
N$22
  Top 0.305: RN5.6 70.12,23.77 70.48,24.13 71.97,24.13 IC2.11 73.73,24.2 74.93,25.4 76,25.4 IC3.7
N$23
  Top 0.254: 71.97,22.86 IC2.10
  Top 0.305: RN5.5 70.92,21.81 IC2.10 73.73,22.93 74.93,24.13 76,24.13 IC3.8
N$24
  Top 2.54: 24.15,73.64 24.15,69.24 20.32,65.41 20.32,46.35
N$25
  Bottom 2.54: 20.32,46.35 20.32,64.77 24.13,68.58 24.13,73.61 24.15,73.64
N$26
  Bottom 2.54: 14.35,60.58 14.35,65.15 19.05,69.85 19.05,73.61 19.07,73.64
N$27
  Bottom 2.54: 26.29,60.58 26.29,64.39 29.21,67.31 29.21,73.61 29.23,73.64
N$28
  Bottom 2.54: 44.07,60.58 44.07,63.12 44.45,63.5 44.45,73.61 44.47,73.64
N$29  (via drill 0.5)
  Top 0.305: R2.C 106.56,33.77 v106.68,33.66 | v106.68,25.4 106.05,26.04 93.73,26.04 93.34,25.65 91.62,25.65 RN2.2
  Bottom 0.305: v106.68,33.66 v106.68,25.4
N$30  (via drill 0.5)
  Top 0.305: R3.C 112.28,33.77 v112.39,33.66 | v112.39,26.04 111.76,26.67 93.47,26.67 93.22,26.42 91.62,26.42 RN2.3
  Bottom 0.305: v112.39,33.66 v112.39,26.04
N$31  (via drill 0.5)
  Top 0.305: R4.C 118,33.77 v118.11,33.66 | v118.11,28.58 116.84,27.3 91.67,27.3 RN2.4
  Bottom 0.305: v118.11,33.66 v118.11,28.58
N$32
  Top 0.305: RN3.8 140.26,32.31 140.97,33.02 140.97,37.98 R8.C
N$42
  Bottom 2.54: 61.85,60.58 61.85,63.88 59.69,66.04 59.69,73.61 59.71,73.64
N$43
  Bottom 2.54: 32.13,60.58 32.13,63.88 34.29,66.04 34.29,73.61 34.31,73.64
N$44
  Bottom 2.54: 38.1,46.35 38.1,64.77 39.37,66.04 39.37,73.61 39.39,73.64
N$45
  Bottom 2.54: 49.91,60.58 49.91,63.12 49.53,63.5 49.53,72.34 49.55,73.64
N$46
  Top 2.54: 49.53,62.87 49.53,73.66 50.16,73.66 50.16,62.87 | 49.53,62.87 50.16,62.87 | 50.16,62.87 50.16,62.23 | 50.16,62.23 50.16,60.32 49.53,60.32 49.53,60.96 | 49.53,60.96 49.53,62.23 | 49.53,62.87 49.53,62.23 | 49.53,62.23 50.16,62.23 | 49.53,60.96 50.8,60.96 | 50.8,60.96 50.8,73.66 48.26,73.66 48.26,59.69 50.8,59.69 50.8,60.96
N$47
  Bottom 2.54: 54.61,73.61 54.63,73.64
N$48
  Bottom 2.54: 55.88,46.35 55.88,63.5 54.61,64.77
N$49
  Top 2.54: 54.61,73.66 54.61,64.77 | 55.88,63.5 55.88,46.35 | 54.61,73.66 55.88,73.66 55.88,64.77 | 55.88,64.77 55.88,63.5 | 55.88,63.5 54.61,64.77 | 54.61,64.77 54.61,45.72 | 54.61,45.72 57.15,45.72 57.15,63.5 55.88,64.77 | 54.61,73.66 53.98,73.66 53.98,45.72 54.61,45.72
N$50
  Top 2.54: 59.05,66.67 59.05,73.66 60.33,73.66 60.33,67.31 62.87,64.77 62.87,59.69 60.96,59.69 60.96,64.14 | 59.05,66.67 60.96,64.77 60.96,64.14 | 59.05,66.67 59.05,66.04 60.96,64.14
N$51
  Top 2.54: 66.67,59.69 66.67,65.41 64.14,67.95 64.14,73.66 65.41,73.66 65.41,68.58 68.58,65.41 68.58,59.69 66.67,59.69
N$52
  Top 2.54: 69.85,73.66 68.58,73.66 68.58,69.85 71.12,67.31 | 71.12,67.31 72.39,66.04 72.39,45.72 74.93,45.72 74.93,64.77 | 74.93,64.77 69.85,69.85 69.85,73.66 | 69.85,73.66 71.12,73.66 71.12,69.22 | 71.12,69.22 71.12,67.31 | 74.93,64.77 74.93,65.41 71.12,69.22
N$53
  Top 2.54: 74.3,73.66 74.3,70.48 78.74,66.04 78.74,59.69 80.64,59.69 80.64,66.04 75.56,71.12 75.56,73.66 74.3,73.66
N$54
  Top 2.54: 45.09,73.66 45.09,59.69 43.18,59.69 43.18,73.66 45.09,73.66
N$55
  Top 2.54: 40.01,73.66 40.01,45.72 37.47,45.72 37.47,64.14 38.73,65.41 38.73,73.66 40.01,73.66
N$56
  Top 2.54: 34.92,73.66 34.92,66.67 33.66,65.41 33.66,59.69 31.11,59.69 31.11,64.77 33.66,67.31 33.66,73.66 34.92,73.66
N$57
  Top 2.54: 29.21,73.66 29.84,73.66 29.84,67.95 27.3,65.41 27.3,59.69 25.4,59.69 25.4,64.77 28.57,67.95 | 29.21,68.58 29.21,73.66 | 29.21,73.66 28.57,73.66 28.57,67.31
N$58
  Top 2.54: 24.77,69.22 24.77,73.66 24.13,73.66 | 24.77,69.22 23.5,67.95 | 23.5,67.95 20.95,65.41 20.95,64.77 | 20.95,64.77 20.95,45.72 19.68,45.72 19.68,65.41 24.13,69.85 24.13,73.66 | 24.13,73.66 23.5,73.66 23.5,67.95 | 24.77,69.22 24.77,68.58 20.95,64.77
N$59
  Top 2.54: 19.68,73.66 19.68,69.85 15.24,65.41 15.24,59.69 13.34,59.69 13.34,64.77 18.41,69.85 18.41,73.66 19.68,73.66
N$60
  Bottom 2.54: 19.05,73.66 18.41,73.66 18.41,69.85 13.34,64.77 13.34,59.69 15.24,59.69 15.24,65.41 19.68,69.85 19.68,73.66
N$61
  Bottom 2.54: 23.5,73.66 23.5,69.22 19.68,65.41 19.68,45.72 20.95,45.72 20.95,64.77 24.77,68.58 24.77,73.66 23.5,73.66
N$62
  Bottom 2.54: 28.57,73.66 28.57,67.95 25.4,64.77 25.4,59.69 27.3,59.69 27.3,65.41 29.84,67.95 29.84,73.66 28.57,73.66
N$63
  Bottom 2.54: 33.66,73.66 33.66,67.31 31.11,64.77 31.11,59.69 33.66,59.69 33.66,65.41 34.92,66.67 34.92,73.66 33.66,73.66
N$64
  Bottom 2.54: 38.73,73.66 38.73,65.41 37.47,64.14 37.47,45.72 40.01,45.72 40.01,73.66 38.73,73.66
N$65
  Bottom 2.54: 45.09,73.66 43.18,73.66 43.18,59.69 45.09,59.69 45.09,73.66
N$66
  Bottom 2.54: 48.26,73.66 48.26,59.69 50.8,59.69 50.8,73.66 48.26,73.66
N$67
  Bottom 2.54: 53.98,73.66 53.98,45.72 57.15,45.72 57.15,63.5 55.88,64.77 55.88,73.66 53.98,73.66
N$68
  Bottom 2.54: 59.05,73.66 59.05,66.04 60.96,64.14 60.96,59.69 62.87,59.69 62.87,64.77 60.33,67.31 60.33,73.66 59.05,73.66
N$69
  Bottom 2.54: 67.69,60.58 67.69,64.39 66.67,65.41 | 66.67,65.41 64.77,67.31 | 64.77,67.31 64.77,73.61 64.79,73.64 | 64.77,67.31 64.14,67.95 64.14,73.66 65.41,73.66 65.41,68.58 68.58,65.41 68.58,59.69 66.67,59.69 66.67,65.41
N$70
  Bottom 2.54: 73.66,46.35 73.66,64.77 72.39,66.04 | 72.39,66.04 69.85,68.58 | 69.85,68.58 69.85,73.61 69.87,73.64 | 69.85,68.58 68.58,69.85 68.58,73.66 71.12,73.66 71.12,69.22 74.93,65.41 74.93,45.72 72.39,45.72 72.39,66.04
N$71
  Bottom 2.54: 79.63,60.58 79.63,65.15 78.74,66.04 | 78.74,66.04 74.93,69.85 | 74.93,69.85 74.93,73.61 74.95,73.64 | 74.93,69.85 74.3,70.48 74.3,73.66 75.56,73.66 75.56,71.12 80.64,66.04 80.64,59.69 78.74,59.69 78.74,66.04
N$81  (via drill 0.5)
  Top 0.305: R7.C 135.14,33.77 v135.25,33.66 | v135.25,31.12 134.62,31.75 92.71,31.75 92.46,31.5 91.62,31.5 RN3.7
  Bottom 0.305: v135.25,33.66 v135.25,31.12
N$82  (via drill 0.5)
  Top 0.305: R6.C 129.43,33.77 v129.54,33.66 | v129.54,30.48 128.91,31.12 93.09,31.12 92.58,30.61 91.71,30.61 RN3.6
  Bottom 0.305: v129.54,33.66 v129.54,30.48
N$83  (via drill 0.5)
  Top 0.305: R5.C 123.71,33.77 v123.83,33.66 | v123.83,29.84 123.19,30.48 93.34,30.48 92.71,29.84 91.67,29.84 RN3.5
  Bottom 0.305: v123.83,33.66 v123.83,29.84
N$89
  Top 0.305: RN5.8 68.52,25.98 69.22,26.67 71.97,26.67 IC2.13 73.73,26.74 74.93,27.94 76,27.94 IC3.5
N$93
  Top 0.305: RN4.6 66.44,21.99 67.31,22.86 67.31,27.3 69.22,29.21 71.97,29.21 IC2.15 73.73,29.28 74.93,30.48 76,30.48 IC3.3
N$94
  Top 0.305: RN4.8 64.84,22.93 66.04,24.13 66.04,28.58 69.22,31.75 71.94,31.75 IC2.17 73.76,31.85 74.93,33.02 76,33.02 IC3.1
N$203
  Top 2.54: X251.2 154.33,69.83 158.12,66.04 K8_B1.COM
N$204
  Top 2.54: X251.3 149.25,68.56 152.4,65.41 152.4,60.83 K8_B1.NC
N$205
  Top 2.54: X251.1 159.41,70.46 163.83,66.04 163.83,60.83 K8_B1.NO
N$206
  Top 2.54: X261.1 144.17,66.65 146.05,64.77 146.05,60.83 K7_B1.NO
N$207
  Top 2.54: X271.1 128.93,60.98 K6_B1.NO
N$208
  Top 2.54: X261.3 134.01,60.94 K7_B1.NC
N$209
  Top 2.54: X261.2 139.09,47.6 K7_B1.COM
N$210
  Top 2.54: X271.3 118.77,66.7 116.84,64.77 116.84,60.83 K6_B1.NC
N$211
  Top 2.54: X271.2 123.85,47.65 K6_B1.COM
N$212
  Top 2.54: X281.3 103.53,69.87 98.42,64.77 98.42,60.96 K5_B1.NC
N$213
  Top 2.54: X281.2 108.61,69.24 104.78,65.41 K5_B1.COM
N$214
  Top 2.54: X281.1 113.69,68.6 110.49,65.41 110.49,60.83 K5_B1.NO
N$215
  Top 2.54: X291.1 74.95,70.46 79.38,66.04 79.38,60.83 K4_B1.NO
N$216
  Top 2.54: X291.3 64.79,67.92 67.31,65.41 67.31,60.96 K4_B1.NC
N$217
  Top 2.54: X291.2 69.87,69.19 73.66,65.41 K4_B1.COM
N$218
  Top 2.54: X301.1 59.71,66.02 61.59,64.14 61.59,60.83 K3_B1.NO
N$219
  Top 2.54: X301.3 49.55,61.57 50.16,60.96 50.16,60.83 K3_B1.NC
N$220
  Top 2.54: X301.2 54.63,47.6 K3_B1.COM
N$221
  Top 2.54: X311.1 44.47,60.98 K2_B1.NO
N$222
  Top 2.54: X311.3 34.31,66.7 32.38,64.77 32.38,60.83 K2_B1.NC
N$223
  Top 2.54: X311.2 39.39,47.65 K2_B1.COM
N$224
  Top 2.54: X3211.1 29.23,67.97 26.04,64.77 26.04,60.83 K1_B1.NO
N$225
  Top 2.54: X3211.3 19.07,69.87 13.97,64.77 13.97,60.96 K1_B1.NC
N$226
  Top 2.54: X3211.2 24.15,69.24 20.32,65.41 K1_B1.COM
N$304
  Top 2.54: 154.33,73.64 154.33,69.19 158.12,65.41 158.12,46.35
N$305
  Top 2.54: 149.25,73.64 149.25,67.92 151.76,65.41 151.76,60.96 152.15,60.58
N$306
  Top 2.54: 159.41,73.64 159.41,70.46 163.83,66.04 163.83,60.83 164.08,60.58
N$307
  Top 2.54: 144.17,73.64 144.17,66.65 146.05,64.77 146.05,60.83 146.3,60.58
N$308
  Top 2.54: 128.93,73.64 128.93,60.98 128.52,60.58
N$309
  Top 2.54: 134.01,73.64 134.01,60.94 134.37,60.58
N$310
  Top 2.54: 139.09,73.64 139.09,47.6 140.34,46.35
N$311
  Top 2.54: 118.77,73.64 118.77,66.7 116.84,64.77 116.84,60.83 116.59,60.58
N$312
  Top 2.54: 123.85,73.64 123.85,47.65 122.56,46.35
N$313
  Top 2.54: 103.53,73.64 103.53,69.87 98.42,64.77 98.42,60.96 98.81,60.58
N$314
  Top 2.54: 108.61,73.64 108.61,69.24 104.78,65.41 104.78,46.35
N$315
  Top 2.54: 113.69,73.64 113.69,67.97 110.49,64.77 110.49,60.83 110.74,60.58
N$360
  Top 2.54: 113.69,73.64 113.69,67.97 111.12,65.41 111.12,60.96 110.74,60.58
N$361
  Top 2.54: 103.53,73.64 103.53,69.87 99.06,65.41 99.06,60.83 98.81,60.58
N$362
  Top 2.54: 108.61,73.64 108.61,68.6 104.78,64.77 104.78,46.35
N$363
  Top 2.54: 128.93,73.64 128.93,60.98 128.52,60.58
N$364
  Top 2.54: 118.77,73.64 118.77,66.7 116.84,64.77 116.84,60.83 116.59,60.58
N$365
  Top 2.54: 123.85,73.64 123.85,47.65 122.56,46.35
N$366
  Top 2.54: 144.17,73.64 144.17,66.02 146.05,64.14 146.05,60.83 146.3,60.58
N$367
  Top 2.54: 134.01,73.64 134.01,60.94 134.37,60.58
N$368
  Top 2.54: 139.09,73.64 139.09,47.6 140.34,46.35
N$369
  Top 2.54: 159.41,73.64 159.41,70.46 163.83,66.04 163.83,60.83 164.08,60.58
N$370
  Top 2.54: 149.25,73.64 149.25,68.56 152.4,65.41 152.4,60.83 152.15,60.58
N$371
  Top 2.54: 154.33,73.64 154.33,69.83 158.12,66.04 158.12,46.35
N$372
  Bottom 2.54: 104.78,46.35 104.78,64.77 108.58,68.58 108.58,73.61 108.61,73.64
N$373
  Bottom 2.54: 98.81,60.58 98.81,65.15 103.5,69.85 103.5,73.61 103.53,73.64
N$374
  Bottom 2.54: 110.74,60.58 110.74,64.39 113.67,67.31 113.67,73.61 113.69,73.64
N$375
  Bottom 2.54: 128.52,60.58 128.52,63.12 128.91,63.5 128.91,73.61 128.93,73.64
N$376
  Bottom 2.54: 146.3,60.58 146.3,63.88 144.15,66.04 144.15,73.61 144.17,73.64
N$377
  Bottom 2.54: 116.59,60.58 116.59,63.88 118.75,66.04 118.75,73.61 118.77,73.64
N$378
  Bottom 2.54: 122.56,46.35 122.56,64.77 123.83,66.04 123.83,73.61 123.85,73.64
N$379
  Bottom 2.54: 134.37,60.58 134.37,63.12 133.99,63.5 133.99,72.34 134.01,73.64
N$380
  Top 2.54: 133.99,62.87 133.99,73.66 134.62,73.66 134.62,62.87 | 133.99,62.87 134.62,62.87 | 134.62,62.87 134.62,62.23 | 134.62,62.23 134.62,60.32 133.99,60.32 133.99,60.96 | 133.99,60.96 133.99,62.23 | 133.99,62.87 133.99,62.23 | 133.99,62.23 134.62,62.23 | 133.99,60.96 135.25,60.96 | 135.25,60.96 135.25,73.66 132.72,73.66 132.72,59.69 135.25,59.69 135.25,60.96
N$381
  Bottom 2.54: 139.09,73.64 139.06,73.61 139.06,64.77 140.34,63.5 140.34,46.99
N$382
  Top 2.54: 139.06,73.66 139.06,64.77 | 139.06,73.66 140.34,73.66 140.34,64.77 141.6,63.5 141.6,45.72 139.06,45.72 | 140.34,63.5 139.06,64.77 | 139.06,64.77 139.06,45.72 | 139.06,73.66 138.43,73.66 138.43,45.72 139.06,45.72
N$383
  Top 2.54: 143.51,73.66 143.51,66.04 145.41,64.14 145.41,59.69 147.32,59.69 147.32,64.77 144.78,67.31 144.78,73.66 143.51,73.66
N$384
  Top 2.54: 151.13,59.69 151.13,65.41 148.59,67.95 148.59,73.66 149.86,73.66 149.86,68.58 153.03,65.41 153.03,59.69 151.13,59.69
N$385
  Top 2.54: 154.31,73.66 153.03,73.66 153.03,69.85 155.57,67.31 | 155.57,67.31 156.84,66.04 156.84,45.72 159.38,45.72 159.38,64.77 | 159.38,64.77 154.31,69.85 154.31,73.66 | 154.31,73.66 155.57,73.66 155.57,69.22 | 155.57,69.22 155.57,67.31 | 159.38,64.77 159.38,65.41 155.57,69.22
N$386
  Top 2.54: 158.75,73.66 158.75,70.48 163.19,66.04 163.19,59.69 165.1,59.69 165.1,66.04 160.02,71.12 160.02,73.66 158.75,73.66
N$387
  Top 2.54: 129.54,73.66 129.54,59.69 127.64,59.69 127.64,73.66 129.54,73.66
N$388
  Top 2.54: 124.46,73.66 124.46,45.72 121.92,45.72 121.92,64.14 123.19,65.41 123.19,73.66 124.46,73.66
N$389
  Top 2.54: 119.38,73.66 119.38,66.67 118.11,65.41 118.11,59.69 115.57,59.69 115.57,64.77 118.11,67.31 118.11,73.66 119.38,73.66
N$390
  Top 2.54: 113.67,73.66 114.3,73.66 114.3,67.95 111.76,65.41 111.76,59.69 109.86,59.69 109.86,64.77 113.03,67.95 | 113.67,68.58 113.67,73.66 | 113.67,73.66 113.03,73.66 113.03,67.31
N$391
  Top 2.54: 109.22,69.22 109.22,73.66 108.58,73.66 | 109.22,69.22 107.95,67.95 | 107.95,67.95 105.41,65.41 105.41,64.77 | 105.41,64.77 105.41,45.72 104.14,45.72 104.14,65.41 108.58,69.85 108.58,73.66 | 108.58,73.66 107.95,73.66 107.95,67.95 | 109.22,69.22 109.22,68.58 105.41,64.77
N$392
  Top 2.54: 104.14,73.66 104.14,69.85 99.69,65.41 99.69,59.69 97.79,59.69 97.79,64.77 102.87,69.85 102.87,73.66 104.14,73.66
N$393
  Bottom 2.54: 103.5,73.66 102.87,73.66 102.87,69.85 97.79,64.77 97.79,59.69 99.69,59.69 99.69,65.41 104.14,69.85 104.14,73.66
N$394
  Bottom 2.54: 107.95,73.66 107.95,69.22 104.14,65.41 104.14,45.72 105.41,45.72 105.41,64.77 109.22,68.58 109.22,73.66 107.95,73.66
N$395
  Bottom 2.54: 113.03,73.66 113.03,67.95 109.86,64.77 109.86,59.69 111.76,59.69 111.76,65.41 114.3,67.95 114.3,73.66 113.03,73.66
N$396
  Bottom 2.54: 118.11,73.66 118.11,67.31 115.57,64.77 115.57,59.69 118.11,59.69 118.11,65.41 119.38,66.67 119.38,73.66 118.11,73.66
N$397
  Bottom 2.54: 123.19,73.66 123.19,65.41 121.92,64.14 121.92,45.72 124.46,45.72 124.46,73.66 123.19,73.66
N$398
  Bottom 2.54: 129.54,73.66 127.64,73.66 127.64,59.69 129.54,59.69 129.54,73.66
N$399
  Bottom 2.54: 132.72,73.66 132.72,59.69 135.25,59.69 135.25,73.66 132.72,73.66
N$400
  Bottom 2.54: 138.43,73.66 138.43,45.72 141.6,45.72 141.6,63.5 140.34,64.77 140.34,73.66 138.43,73.66
N$401
  Bottom 2.54: 143.51,73.66 143.51,66.04 145.41,64.14 145.41,59.69 147.32,59.69 147.32,64.77 144.78,67.31 144.78,73.66 143.51,73.66
N$402
  Bottom 2.54: 152.15,60.58 152.15,64.39 151.13,65.41 | 151.13,65.41 149.22,67.31 | 149.22,67.31 149.22,73.61 149.25,73.64 | 149.22,67.31 148.59,67.95 148.59,73.66 149.86,73.66 149.86,68.58 153.03,65.41 153.03,59.69 151.13,59.69 151.13,65.41
N$403
  Bottom 2.54: 158.12,46.35 158.12,64.77 156.84,66.04 | 156.84,66.04 154.31,68.58 | 154.31,68.58 154.31,73.61 154.33,73.64 | 154.31,68.58 153.03,69.85 153.03,73.66 155.57,73.66 155.57,69.22 159.38,65.41 159.38,45.72 156.84,45.72 156.84,66.04
N$404
  Bottom 2.54: 164.08,60.58 164.08,65.15 163.19,66.04 | 163.19,66.04 159.38,69.85 | 159.38,69.85 159.38,73.61 159.41,73.64 | 159.38,69.85 158.75,70.48 158.75,73.66 160.02,73.66 160.02,71.12 165.1,66.04 165.1,59.69 163.19,59.69 163.19,66.04
OC_R1  (via drill 0.5)
  Top 0.305: RN2.8 89.95,24.89 88.77,24.89 88.14,24.26 IC3.11 85.8,24.13 v83.82,24.13 | K8_B1.C1 164.08,44.07 161.29,41.27 92.71,41.27 v90.81,39.37
  Bottom 0.305: v90.81,39.37 90.81,33.66 83.82,26.67 v83.82,24.13
OC_R2  (via drill 0.5)
  Top 0.305: RN2.7 89.99,25.65 88.39,25.65 88.27,25.53 IC3.12 85.8,25.4 v82.55,25.4 | K7_B1.C1 146.3,44.07 144.15,41.91 91.44,41.91 v88.9,39.37
  Bottom 0.305: v88.9,39.37 88.9,33.66 82.55,27.3 v82.55,25.4
OC_R3  (via drill 0.5)
  Top 0.305: RN2.6 89.99,26.42 88.52,26.42 88.14,26.8 IC3.13 81.53,26.8 81.41,26.67 v81.28,26.67 | K6_B1.C1 128.52,44.7 126.36,42.55 90.17,42.55 v87,39.37
  Bottom 0.305: v87,39.37 87,33.66 81.28,27.94 v81.28,26.67
OC_R4  (via drill 0.5)
  Top 0.305: RN2.5 89.94,27.3 88.9,27.3 88.14,28.07 IC3.14 85.8,27.94 v80.01,27.94 | K5_B1.C1 110.74,44.7 109.22,43.18 88.9,43.18 v85.09,39.37
  Bottom 0.305: v85.09,39.37 85.09,33.66 80.01,28.58 v80.01,27.94
OC_R5  (via drill 0.5)
  Top 0.305: RN3.4 89.94,29.84 88.9,29.84 88.39,29.34 IC3.15 85.8,29.46 79.63,29.46 v79.38,29.21 | K4_B1.C1 79.63,42.93 v83.19,39.37
  Bottom 0.305: v83.19,39.37 83.19,33.02 v79.38,29.21
OC_R6  (via drill 0.5)
  Top 0.305: RN3.3 89.9,30.61 IC3.16 85.8,30.73 79.63,30.73 79.38,30.48 v78.74,30.48 | K3_B1.C1 61.85,44.83 62.87,43.81 76.83,43.81 v81.28,39.37
  Bottom 0.305: v81.28,39.37 81.28,32.38 79.38,30.48 v78.74,30.48
OC_R7  (via drill 0.5)
  Top 0.305: RN3.2 89.99,31.5 88.52,31.5 88.14,31.88 IC3.17 85.8,31.75 v78.11,31.75 | K2_B1.C1 44.07,44.2 44.45,43.81 61.59,43.81 62.23,43.18 75.56,43.18 v79.38,39.37
  Bottom 0.305: v79.38,39.37 79.38,34.92 80.01,34.29 80.01,32.38 79.38,31.75 v78.11,31.75
OC_R8  (via drill 0.5)
  Top 0.305: RN3.1 89.95,32.26 88.9,32.26 88.01,33.15 IC3.18 84.2,33.15 84.07,33.02 v78.74,33.02 | K1_B1.C1 26.29,44.2 27.3,43.18 61.21,43.18 61.85,42.55 74.3,42.55 v77.47,39.37
  Bottom 0.305: v77.47,39.37 77.47,34.92 v78.74,33.02
REG_5V  (via drill 0.5, 0.9)
  Top 0.254: RN6.6 RN6.5 47.23,29.59 47.75,29.59 48.13,29.97 v48.51,29.97 | 44.98,24.41 45.09,24.51
  Top 0.305: H1.1 7.46,19.27 4.95,16.76 4.95,15.83 RNB.6 | 59.05,31.75 59.05,34.92 v58.42,35.56 | 59.05,31.75 59.05,27.94 60.2,26.8 IC2.6 | R1.A 102.35,39.48 102.87,40.01 107.95,40.01 | 107.95,40.01 113.67,40.01 | 113.67,40.01 119.38,40.01 | 119.38,40.01 125.09,40.01 | 125.09,40.01 130.81,40.01 | 130.81,40.01 136.53,40.01 | 136.53,40.01 141.6,40.01 142.24,39.37 142.24,38.22 R8.A | R7.A 136.64,39.89 136.53,40.01 | R6.A 130.93,39.89 130.81,40.01 | R5.A 125.21,39.89 125.09,40.01 | R4.A 119.5,39.89 119.38,40.01 | R3.A 113.78,39.89 113.67,40.01 | R2.A 108.06,39.89 107.95,40.01 | 56.52,31.75 59.05,31.75
  Top 0.406: v1.91,18.41 4.45,20.95 7.37,20.95 H1.1 | U$18.A3 U$18.A2 U$18.A1 | IC2.18 70.36,33.15 69.85,33.66 69.85,37.11 CB3.2 CA3.2 67.29,35.54 v66.67,34.92 | 62.71,26.67 IC2.6
  Top 0.61: CA1.2 44.98,24.41 | 45.09,24.51 45.09,24.77 48.51,28.19 v48.51,29.97
  Top 0.813: 16.13,20.83 9.96,20.83 H1.1 | 16.13,20.83 17.27,20.83 18.41,19.69 20.75,19.69 C4.1 | IC1.4 16.13,19.15 16.13,20.83 | IC2.18 73.15,33.15 73.66,33.66 73.66,34.29 74.3,34.92 88.9,34.92 93.34,39.37 97.16,39.37 | 97.16,39.37 102.23,39.37 102.35,39.48 | C1.+ 96.77,38.99 97.16,39.37
  Top 1.016: H1.1 9.27,18.41 9.27,17.65 9.4,17.53 9.4,5.59 13.46,1.52 37.72,1.52 38.73,2.54 38.73,6.35 39.37,6.99 44.83,6.99 v45.09,7.24 45.21,7.37 | 22.05,19.69 22.23,19.69 22.86,20.32 22.86,26.67 v20.32,29.21 | X1.2 45.09,22.25 CA1.2
  Top 1.27: 20.75,19.69 22.05,19.69
  Bottom 0.254: v1.91,18.41 1.91,24.13 3.17,25.4 U$18.A3
  Bottom 0.406: v66.67,34.92 59.05,34.92 v58.42,35.56
  Bottom 0.61: FOR_NANO.5V 50.29,31.75 v48.51,29.97
  Bottom 1.016: v45.09,7.24 X1.2
REG_12V  (via drill 0.5)
  Top 0.61: IC1.7 13.46,23.16 | 14.1,22.48 14.15,22.48
  Top 0.813: v18.41,22.48 14.15,22.48 13.46,23.16 | v25.4,22.48 26.04,21.84 C3.1 26.04,14.61 27.3,13.34 BRA1.+
  Bottom 0.813: v18.41,22.48 v25.4,22.48
UNREG_12V  (via drill 0.5, 0.9)
  Top 0.762: v95.38,22.99 IC3.10
  Top 2.54: X2.2 26.97,7.32 21.59,12.7 BRA1.~@1 21.59,15.24 | 21.59,15.24 BRA1.~@2 | U$1.TIP 15.14,13.87 16.51,15.24 21.59,15.24
  Bottom 1.27: 98.81,42.55 98.81,26.42 v95.38,22.99
  Bottom 1.676: K1_B1.C2 14.35,44.2 | K2_B1.C2 32.13,43.43 | K3_B1.C2 49.91,42.93 | 67.69,42.93 K4_B1.C2 67.69,42.8 67.94,42.55 98.81,42.55 K5_B1.C2 98.81,42.8 99.06,42.55 116.59,42.55 K6_B1.C2 116.59,42.8 116.84,42.55 134.37,42.55 K7_B1.C2 134.37,42.8 134.62,42.55 151.13,42.55 | 151.13,42.55 152.15,42.55 K8_B1.C2 | C2.+ 151.13,42.55 | v27.94,31.75 27.94,41.91 28.57,42.55
  Bottom 1.778: 33.02,42.55 49.53,42.55 49.91,42.93 50.29,42.55 67.31,42.55 67.69,42.93 | 33.02,42.55 28.57,42.55 16,42.55 14.35,44.2 | 32.13,43.43 33.02,42.55 | v27.94,31.75 27.94,5.44 X2.2

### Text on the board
tNames: NC | COM | NO | NC | COM | NO | NC | COM | NO | NC | COM | NO | NC | COM | NO | NC | COM | NO | NC | COM | NO | NC | COM | NO | 1 | 4 | 5 | 8 | Bank 1 | A0 | A1 | A2 | Address | SC | SCL | SDA | +5V | GND | 2016 ControlEverything.com | MCP23008 | ANSR8G5LE | REV.E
